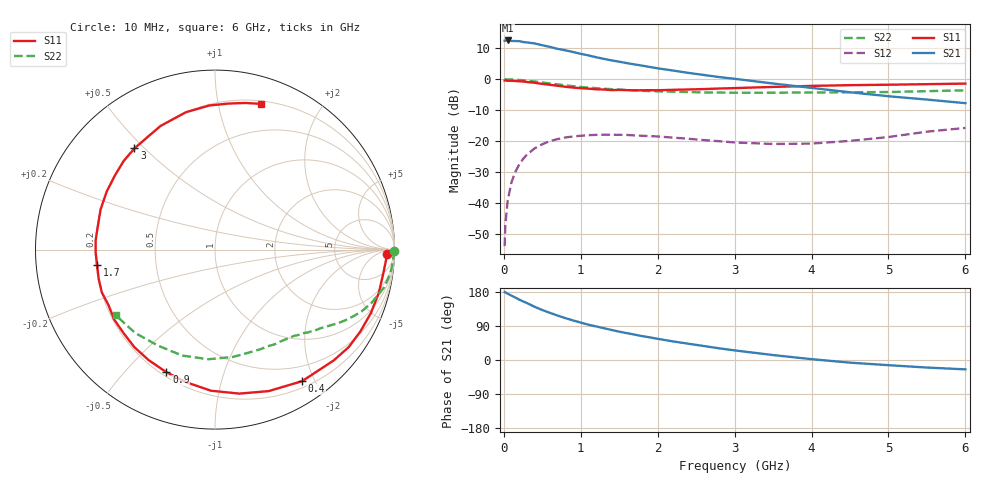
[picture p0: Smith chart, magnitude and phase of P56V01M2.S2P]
! SIEMENS Small Signal Semiconductors
! BFP183
! Si NPN RF Bipolar Junction Transistor in SOT143
! VCE = 6 V  IC = 1.2 mA
! Common Emitter S-Parameters:  March  1996
# GHz  S  MA  R  50
!  f  S11  S21  S12  S22
! GHz  MAG  ANG  MAG  ANG  MAG  ANG  MAG  ANG
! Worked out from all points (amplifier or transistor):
!   36 points, 10 MHz to 6 GHz, reference 50 ohm
!   highest |S21| = 12.6 dB at 50 MHz (marker M1)
!   |S21| within 3 dB of that: start of sweep to 759.3 MHz
!   unconditionally stable (mu >= 1): 2.438 GHz to end of sweep
!   at 250 MHz: K = 0.10, MSG = 18.9 dB, |S12| = -25.8 dB
!   at 1.4 GHz: K = 0.56, MSG = 12.0 dB, |S12| = -17.9 dB
!   at 6 GHz: K = 1.01, MAG = 3.3 dB, |S12| = -15.7 dB
!   S11 on the Smith chart (normalised r, x): 10 MHz: 35, -19; 400 MHz: 0.28, -1.83; 900 MHz: 0.22, -0.66; 1.7 GHz: 0.20, -0.06; 3 GHz: 0.20, +0.47; 6 GHz: 0.23, +1.34
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0.01  0.9571 -1.4  4.202 179.3  0.002 84.7  0.9999 -0.5
0.02  0.956 -2.9  4.215 178.5  0.0045 85.5  0.9992 -1.1
0.05  0.9478 -7.4  4.249 174.9  0.0109 87.2  0.9943 -2.5
0.1  0.9442 -14.7  4.167 169.9  0.0218 80.6  0.9909 -5.1
0.15  0.9379 -22.1  4.157 164.7  0.0319 76.6  0.9855 -7.7
0.2  0.9298 -29.3  4.137 159.4  0.042 72.8  0.9751 -10.1
0.4  0.8792 -56.5  3.8 140.4  0.0763 57.5  0.921 -18.8
0.5  0.8433 -69.2  3.558 131.9  0.0891 50.1  0.8877 -22.7
0.6  0.8137 -80.4  3.339 124.3  0.1001 44.1  0.8572 -25.6
0.7  0.7866 -91.6  3.104 117.2  0.1081 38.4  0.8266 -28.4
0.8  0.7565 -102.1  2.944 110.5  0.1145 33.6  0.8009 -30.7
0.9  0.7349 -111.6  2.764 104.4  0.119 29.1  0.7736 -32.9
1.1  0.7051 -129.6  2.432 93.1  0.1249 21.5  0.733 -36.7
1.4  0.6691 -152.4  2.024 79.3  0.1272 12.4  0.6932 -41.8
1.7  0.6625 -172.4  1.742 67.0  0.1236 6.4  0.6591 -46.5
2.2  0.6756 160.7  1.385 49.0  0.1139 0.2  0.6289 -54.4
2.6  0.6944 143.2  1.175 36.9  0.104 -1.2  0.6128 -61.6
3  0.7207 128.5  1.019 25.4  0.0951 0.1  0.6054 -69.6
3.5  0.7527 113.8  0.855 13.0  0.0899 6.6  0.6064 -80.4
4.5  0.8038 92.2  0.617 -7.0  0.1009 21.6  0.618 -107.2
5.5  0.8345 78.2  0.47 -19.9  0.1422 26.8  0.643 -133.8
6  0.8521 72.3  0.411 -24.7  0.1636 23.9  0.6632 -146.5
